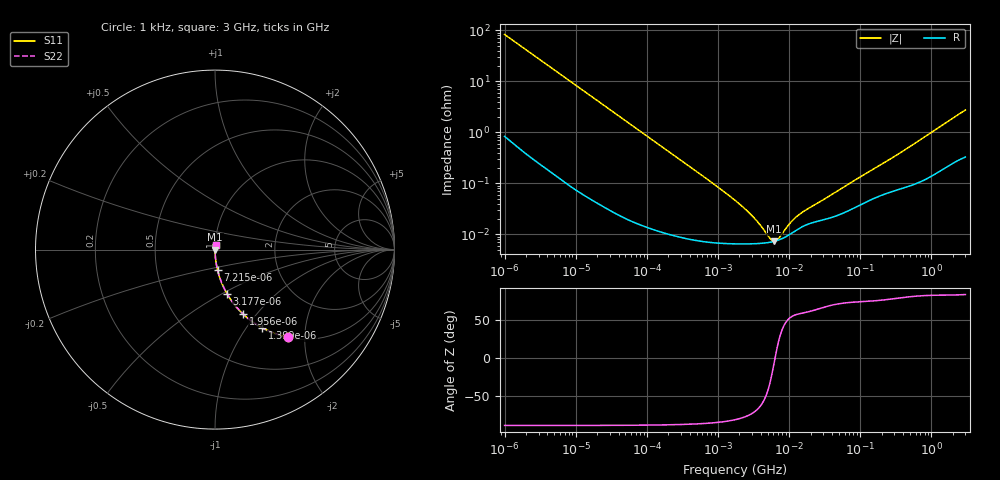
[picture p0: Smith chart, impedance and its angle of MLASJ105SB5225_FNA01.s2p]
! MLASJ105SB5225_FNA01  S-PARAMETER MODEL  ( Standard Model )
! Model Generated by TAIYO YUDEN Corporation (http://www.ty-top.com)
! Version 2.0
! TAIYO YUDEN Control No. 240725
! Copyright(c) 2007 TAIYO YUDEN CO.,LTD. All Rights Reserved.
! Product Description (link to TY-COMPAS)
! https://ds.yuden.co.jp/TYCOMPAS/or/detail?pn=MLASJ105SB5225KFNA01&u=M
! Products Name : Multilayer Ceramic Capacitors
! Characteristics :
!  Capacitance : 2.2 [uF] , Rated Voltage : 6.3 [V] , TCC : X5R
!  Case Size : 1.0 x 0.5 / 0.039 x 0.02 [mm/inch] , Thickness : 0.5 / 0.02 [mm/inch]
!  (Conditions: Temperature = 25 [degC] , DC Bias Voltage = 0 [V])
! External Node Assignments :
!  1  o---| |---o  2
! GND o---------o GND
! Frequency Range : 1kHz  -  3GHz  [ 401 STEP ]
# MHZ S RI R 50
! Freq[MHz].  S11 Real  S11 Imag  S21 Real  S21 Imag  S12 Real  S12 Imag  S22 Real  S22 Imag
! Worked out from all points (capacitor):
!   401 points, 1 kHz to 3 GHz, reference 50 ohm
!   read as one part in series: C = 1.91 uF near 1.077 kHz
!   lowest |Z| = 7.36 mohm at 6.153 MHz (marker M1)
!   series resonance near 6.352 MHz, so ESL is about 330 pH
!   S11 on the Smith chart (normalised r, x): 1 kHz: 1.02, -1.66; 1.399 kHz: 1.01, -1.19; 1.956 kHz: 1.01, -0.85; 3.177 kHz: 1.00, -0.53; 7.215 kHz: 1.00, -0.23; 3 GHz: 1.01, +0.05
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0.001  0.4092 -0.4867  0.5908 0.4867  0.5908 0.4867  0.4092 -0.4867
0.001399  0.2636 -0.4358  0.7364 0.4358  0.7364 0.4358  0.2636 -0.4358
0.001956  0.1561 -0.3584  0.8439 0.3584  0.8439 0.3584  0.1561 -0.3584
0.003177  0.0667 -0.2451  0.9333 0.2451  0.9333 0.2451  0.0667 -0.2451
0.007215  0.0143 -0.1146  0.9857 0.1146  0.9857 0.1146  0.0143 -0.1146
0.01216  0.00538 -0.0688  0.9946 0.0688  0.9946 0.0688  0.00538 -0.0688
0.033275  0.00092 -0.0254  0.9991 0.0254  0.9991 0.0254  0.00092 -0.0254
0.147855  0.000148 -0.00577  0.9999 0.00577  0.9999 0.00577  0.000148 -0.00577
0.762639  7.1e-05 -0.00111  0.9999 0.00111  0.9999 0.00111  7.1e-05 -0.00111
1.732051  6.56e-05 -0.000462  0.9999 0.000462  0.9999 0.000462  6.56e-05 -0.000462
3.03007  6.56e-05 -0.000221  0.9999 0.000221  0.9999 0.000221  6.56e-05 -0.000221
4.739869  6.84e-05 -8.15e-05  0.9999 8.15e-05  0.9999 8.15e-05  6.84e-05 -8.15e-05
5.30084  7e-05 -5e-05  0.9999 5e-05  0.9999 5e-05  7e-05 -5e-05
6.153411  7.31e-05 -8.72e-06  0.9999 8.72e-06  0.9999 8.72e-06  7.31e-05 -8.72e-06
7.414467  7.94e-05 4.24e-05  0.9999 -4.24e-05  0.9999 -4.24e-05  7.94e-05 4.24e-05
7.988506  8.3e-05 6.29e-05  0.9999 -6.29e-05  0.9999 -6.29e-05  8.3e-05 6.29e-05
10.37087  0.000102 0.000134  0.9999 -0.000134  0.9999 -0.000134  0.000102 0.000134
12.49624  0.00012 0.000183  0.9999 -0.000183  0.9999 -0.000183  0.00012 0.000183
15.62917  0.000144 0.000237  0.9999 -0.000237  0.9999 -0.000237  0.000144 0.000237
21.06097  0.000169 0.000315  0.9998 -0.000315  0.9998 -0.000315  0.000169 0.000315
256.0921  0.000672 0.00285  0.9993 -0.00285  0.9993 -0.00285  0.000672 0.00285
3000  0.00401 0.0271  0.996 -0.0271  0.996 -0.0271  0.00401 0.0271
